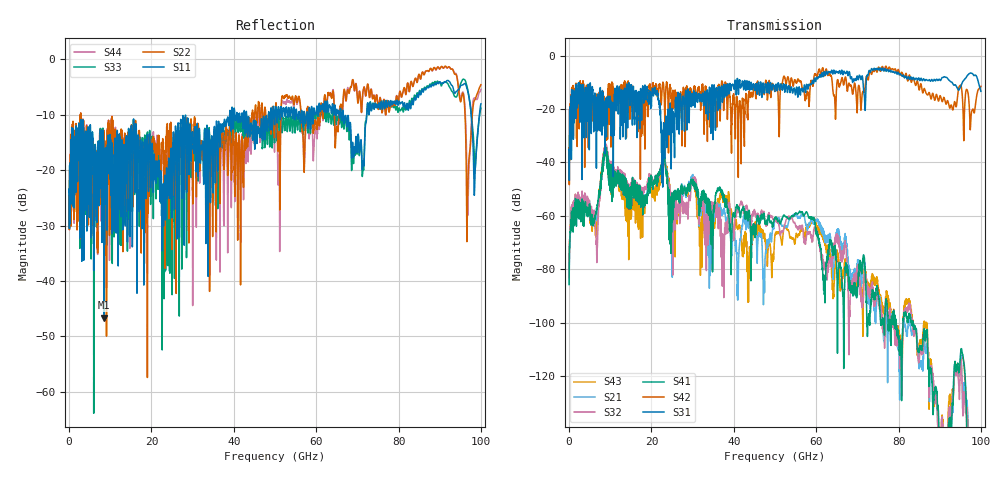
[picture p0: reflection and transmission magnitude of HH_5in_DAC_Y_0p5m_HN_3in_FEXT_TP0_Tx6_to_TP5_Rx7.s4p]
# GHz S RI R 45
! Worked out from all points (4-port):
!   4000 points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, 25 MHz to 100 GHz, reference 45 ohm
!   strongest paths, dB at 25 MHz, 25.02 GHz, 50.02 GHz, 75.03 GHz, 100 GHz:
!     S31: -35.3, -22.0, -12.5, -4.7, -13.3
!     S42: -34.9, -18.5, -12.5, -4.7, -11.5
!     S41: -85.7, -53.4, -60.9, -89.3, -170.6
!     S32: -83.0, -63.0, -61.4, -91.0, -178.7
!     S21: -85.6, -55.6, -61.0, -90.1, -174.5
!     S43: -81.8, -55.1, -67.3, -86.7, -173.5
!   lowest |S11| = -46.6 dB at 8.45 GHz (marker M1), VSWR 1.01, Z = 44.7 - j0.276 ohm
!   |S11| at or under -10 dB: start of sweep to 38.99 GHz; 43.12 GHz to 48.4 GHz (5.275 GHz wide, 11.5 % of centre); 66.6 GHz to 72.29 GHz (5.688 GHz wide, 8.19 % of centre)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
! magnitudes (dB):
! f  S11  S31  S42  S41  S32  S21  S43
! 25 MHz  -23.9  -35.3  -34.9  -85.7  -83.0  -85.6  -81.8
! 6.775 GHz  -29.4  -22.5  -20.1  -57.2  -74.4  -60.3  -63.1
! 8.45 GHz  -46.6  -19.8  -16.6  -36.4  -35.2  -36.0  -35.0
! 14.18 GHz  -28.4  -16.4  -10.2  -54.7  -51.5  -53.5  -60.8
! 38.42 GHz  -10.8  -11.7  -23.3  -57.1  -63.9  -61.5  -54.3
! 43.73 GHz  -11.9  -9.7  -14.3  -58.4  -58.6  -62.5  -81.6
! 100 GHz  -8.0  -13.3  -11.5  -170.6  -178.7  -174.5  -173.5
